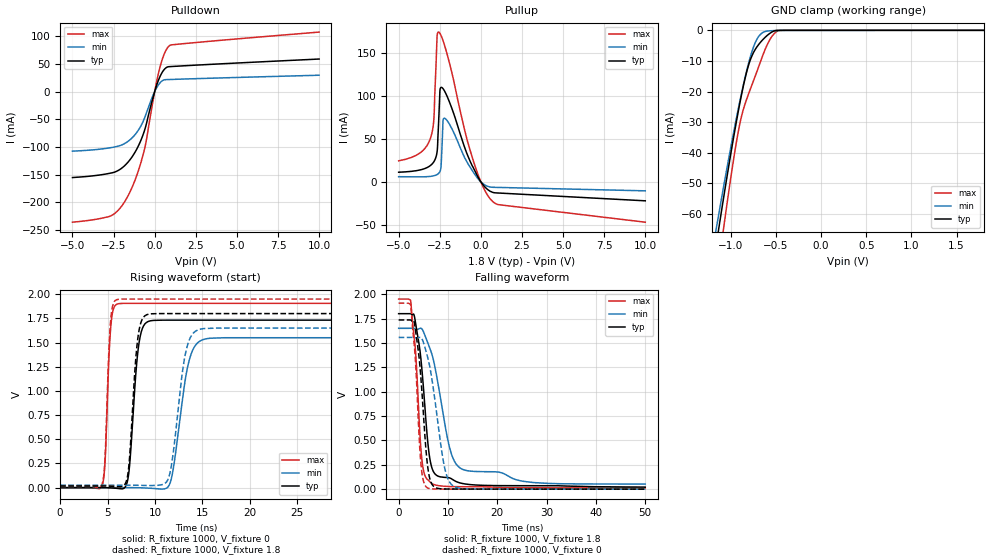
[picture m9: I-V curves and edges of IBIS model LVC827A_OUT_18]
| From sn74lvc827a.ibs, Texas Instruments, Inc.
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[Model]   LVC827A_OUT_18
Model_type  3-state
Enable   Active-Low
Vref =   0
Rref =   1000
Cref =   30p
Vmeas =   0.9
| variable   typ   min   max
C_comp   6.12pF   5.54pF   6.96pF
| C_pullup   7.31pF   6.55pF   7.90pF
| C_pulldown   9.71pF   6.91pF   14.43pF
| C_tri-state   6.12pF   5.54pF   6.96pF
[Temperature Range]   40   100   -40
| Ambient temperature   25   85   -40
[Voltage range]   1.8   1.65   1.95
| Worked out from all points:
|   slope of the pulldown table from 0 to 0.27 V, typ, clamps not added: 11.5 ohm
|   slope of the pullup table from 0 to 0.27 V, typ, clamps not added: 41.6 ohm
|   GND clamp passes 1 mA (typ) near -0.57 V on its own axis
|   rising waveform, R_fixture 1000, V_fixture 0: 20-80 % time 756ps typ, 1.32ns min, 447ps max; typ from 0 V to 1.73 V
|   falling waveform, R_fixture 1000, V_fixture 1.8: 20-80 % time 1.88ns typ, 3.61ns min, 1.39ns max; typ from 1.8 V to 0.021 V
|   rising waveform, R_fixture 1000, V_fixture 1.8: 20-80 % time 709ps typ, 1.18ns min, 434ps max; typ from 0.017 V to 1.8 V
|   falling waveform, R_fixture 1000, V_fixture 0: 20-80 % time 1.58ns typ, 2.63ns min, 1.26ns max; typ from 1.74 V to 0 V
[GND Clamp]
| LVC827A_OUT_18
|   Voltage   I(typ)   I(min)   I(max)
-5V       -931.5mA   -844.2mA   -1.078A
-1.17V    -72.22mA   -66.78mA   -84.97mA
-1.135V   -65.53mA   -60.79mA   -77.21mA
-1.07V    -53.37mA   -49.89mA   -63.11mA
-915mV    -26.52mA   -25.66mA   -33.14mA
-865mV    -19.06mA   -18.67mA   -26.5mA
-800mV    -11.29mA   -10.64mA   -20.68mA
-740mV    -6.897mA   -4.951mA   -15.96mA
-675mV    -4.109mA   -1.476mA   -10.71mA
-585mV    -1.43mA    -210uA     -4.111mA
-500mV    -61.85uA   -75.56uA   -604uA
1.8V      48.72pA    12.03nA    -889pA
[Pulldown]
| LVC827A_OUT_18
|   Voltage   I(typ)   I(min)   I(max)
-5V       -155.4mA   -107.6mA   -236.1mA
-2.675V   -147.3mA   -101.4mA   -224.7mA
-2.165V   -141.6mA   -98.13mA   -212.7mA
-1.67V    -129.1mA   -90.89mA   -191.1mA
-1.19V    -109.2mA   -77.65mA   -159.6mA
-760mV    -82.21mA   -57.51mA   -120.1mA
-530mV    -61.24mA   -40.76mA   -91.59mA
-5mV      -517.7uA   -324.8uA   -814.3uA
255mV     22.46mA    13.33mA    36.36mA
575mV     39.79mA    21.17mA    67.62mA
895mV     45.13mA    21.85mA    82.9mA
10V       58.88mA    29.61mA    107.6mA
[Pullup]
| LVC827A_OUT_18
|   Voltage   I(typ)   I(min)   I(max)
-5V       11.23mA    6.027mA    24.52mA
-3.04V    19.47mA    6.491mA    52.16mA
-2.86V    23.37mA    7.129mA    72.44mA
-2.665V   34.58mA    8.542mA    168.3mA
-2.565V   70.93mA    9.98mA     174.1mA
-2.48V    107.5mA    12.39mA    172.4mA
-2.415V   109.9mA    19.64mA    169.9mA
-2.3V     108.4mA    71.43mA    164.1mA
-2.205V   105.5mA    74mA       158.6mA
-520mV    18.56mA    13.07mA    28.33mA
715mV     -12.14mA   -6.269mA   -22.75mA
10V       -22mA      -10.39mA   -46.85mA
[Ramp]
| LVC827A_OUT_18
| variable   typ   min   max
dV/dt_r   1.05/7.64E-10   0.94/1.33E-09   1.15/4.55E-10
dV/dt_f   1.07/1.88E-09   0.96/3.61E-09   1.16/1.39E-09
R_load = 1000
[Rising Waveform]
| LVC827A_OUT_18
R_fixture =   1000
C_fixture =   0
L_fixture =   0
V_fixture =   0
V_fixture_min = 0
V_fixture_max = 0
|   Time   V(typ)   V(min)   V(max)
0s        484.9pV    3.083nV    17.23nV
4.45ns    299.3uV    284.6uV    26.8mV
5.325ns   -2.66mV    279uV      1.651V
6.005ns   -7.475mV   278.6uV    1.898V
7.15ns    94.11mV    273.3uV    1.905V
8.24ns    1.445V     -686.7uV   1.906V
9.295ns   1.719V     -5.005mV   1.906V
11.6ns    1.732V     50.65mV    1.906V
14.99ns   1.732V     1.528V     1.906V
50ns      1.732V     1.55V      1.906V
[Falling Waveform]
| LVC827A_OUT_18
R_fixture =   1000
C_fixture =   0
L_fixture =   0
V_fixture =   1.8
V_fixture_min = 1.65
V_fixture_max = 1.95
|   Time   V(typ)   V(min)   V(max)
0s        1.8V       1.65V      1.95V
2.405ns   1.8V       1.65V      1.939V
3.195ns   1.773V     1.649V     1.54V
4.745ns   1.211V     1.642V     289mV
5.885ns   493mV      1.504V     97.22mV
6.605ns   243.5mV    1.405V     63.2mV
10.32ns   115.7mV    429.4mV    27.1mV
12.57ns   62.42mV    213.7mV    25.32mV
27.37ns   35.41mV    67.77mV    15.05mV
50ns      21.12mV    52.57mV    12.12mV
[Rising Waveform]
| LVC827A_OUT_18
R_fixture =   1000
C_fixture =   0
L_fixture =   0
V_fixture =   1.8
V_fixture_min = 1.65
V_fixture_max = 1.95
|   Time   V(typ)   V(min)   V(max)
0s        17.42mV    25.58mV    11.98mV
4.45ns    17.6mV     25.74mV    44.91mV
5.295ns   15.02mV    25.67mV    1.695V
5.93ns    12.24mV    25.63mV    1.942V
7.11ns    123.7mV    25.55mV    1.95V
8.145ns   1.512V     24.74mV    1.95V
9.12ns    1.788V     22.2mV     1.95V
11.45ns   1.8V       107.1mV    1.95V
14.51ns   1.8V       1.631V     1.95V
50ns      1.8V       1.65V      1.95V
[Falling Waveform]
| LVC827A_OUT_18
R_fixture =   1000
C_fixture =   0
L_fixture =   0
V_fixture =   0
V_fixture_min = 0
V_fixture_max = 0
|   Time   V(typ)   V(min)   V(max)
0s        1.736V     1.557V     1.908V
2.435ns   1.735V     1.557V     1.889V
3.38ns    1.645V     1.553V     1.338V
4.495ns   1.15V      1.555V     273.1mV
4.99ns    796mV      1.51V      92.57mV
5.72ns    306mV      1.383V     17.72mV
6.755ns   50.31mV    1.125V     3.067mV
9.215ns   2.063mV    247mV      1.029mV
11.14ns   1.534mV    30.62mV    894.2uV
50ns      141.6uV    234.4uV    18.98uV
